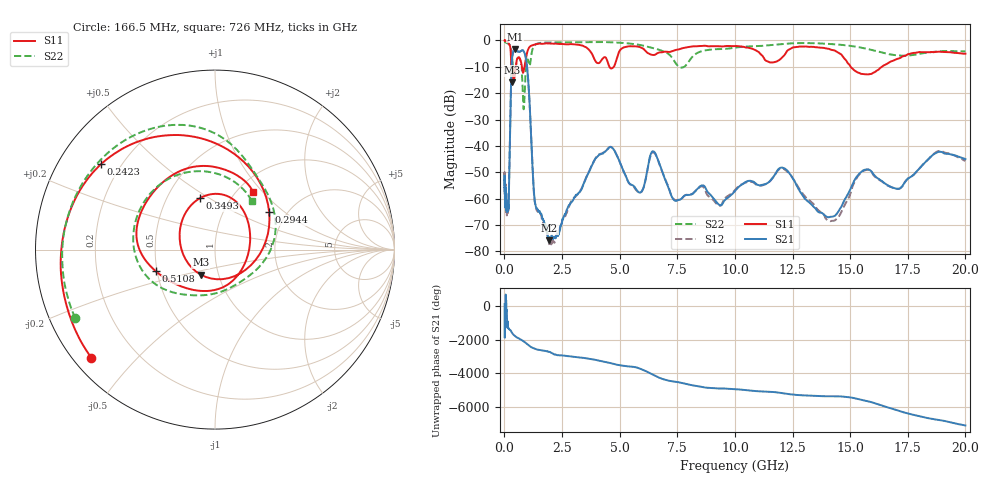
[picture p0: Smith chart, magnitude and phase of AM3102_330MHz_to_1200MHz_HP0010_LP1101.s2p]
! Date/Time: Tue, Sep 11, 2018 5:11 PM
! Network Analyzer: Agilent Technologies E8362B Rev: A.07.50.63
! Sweep from 0.010 to 20.000 GHz, 1601 Points, Sweep Type: LOG
! Power Supply: 4.949 V, 0.001 A
# Hz S DB R 50
!freq MagS11 AngS11 MagS21 AngS21 MagS12 AngS12 MagS22 AngS22
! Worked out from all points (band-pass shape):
!   1601 points, 10 MHz to 20 GHz, reference 50 ohm
!   highest |S21| = -3.26 dB at 464.5 MHz (marker M1); lowest = -75.8 dB at 1.95 GHz (marker M2)
!   |S21| within 3 dB of the highest: 340.5 MHz to 923.4 MHz (582.9 MHz wide, 92.2 % of centre)
!   lowest |S11| = -15.9 dB at 319.2 MHz (marker M3), VSWR 1.38, Z = 41.1 - j11.7 ohm
!   |S11| at or under -10 dB: 298 MHz to 500.2 MHz (202.2 MHz wide, 50.7 % of centre); 4.558 GHz to 4.745 GHz (187.2 MHz wide, 4.02 % of centre); 15.03 GHz to 16.37 GHz (1.348 GHz wide, 8.59 % of centre)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
!   |S22| runs from -26.1 to -0.3 dB; largest |S21 - S12| = 0.012
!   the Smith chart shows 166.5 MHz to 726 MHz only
!   S11 on the Smith chart (normalised r, x): 166.5 MHz: 0.05, -0.38; 242.3 MHz: 0.13, +0.33; 294.4 MHz: 1.63, +0.79; 349.3 MHz: 0.72, +0.46; 510.8 MHz: 0.49, -0.14; 726 MHz: 1.17, +0.89
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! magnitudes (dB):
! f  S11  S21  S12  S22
! 10 MHz  0.0  -55.8  -50.0  -0.3
! 35.55 MHz  0.0  -61.3  -60.2  -0.6
! 126.4 MHz  -0.4  -65.1  -64.4  -1.1
! 166.5 MHz  -0.8  -64.3  -64.4  -1.2
! 242.3 MHz  -2.0  -36.6  -36.7  -1.8
! 294.4 MHz  -8.7  -14.5  -14.6  -3.4
! 319.2 MHz  -15.9  -8.4  -8.4  -5.6
! 349.3 MHz  -10.5  -5.7  -5.8  -7.7
! 447.2 MHz  -13.4  -3.3  -3.3  -12.3
! 464.5 MHz  -12.6  -3.3  -3.3  -11.5
! 510.8 MHz  -9.1  -3.5  -3.6  -8.9
! 726 MHz  -8.3  -4.0  -4.0  -9.4
! 837.2 MHz  -11.7  -4.1  -4.1  -26.1
! 984 MHz  -4.7  -10.1  -10.1  -7.6
! 1.302 GHz  -1.6  -59.6  -60.3  -1.9
! 1.59 GHz  -1.3  -65.8  -65.9  -0.9
! 1.95 GHz  -1.2  -75.8  -77.3  -0.8
! 4.5 GHz  -8.6  -41.0  -40.9  -0.6
! 5.652 GHz  -2.2  -55.6  -55.9  -1.4
! 12.09 GHz  -6.1  -48.3  -48.6  -1.3
! 14.14 GHz  -3.4  -66.9  -68.6  -1.3
! 20 GHz  -5.0  -45.0  -45.8  -4.2
